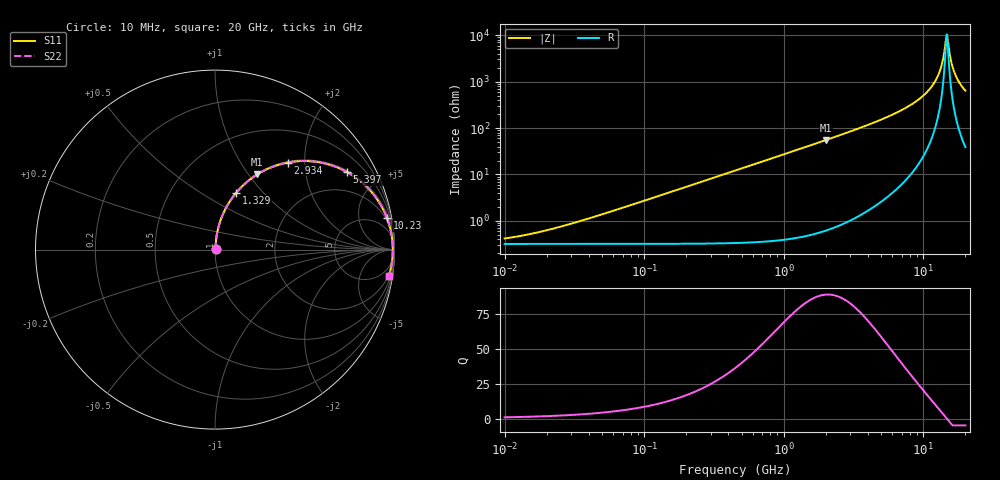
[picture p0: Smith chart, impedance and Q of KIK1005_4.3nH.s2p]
!version-3
!date-01.2023
!Series
# Hz S RI R 50
!Freq ReS11 ImS11 ReS21 ImS21 ReS12 ImS12 ReS22 ImS22
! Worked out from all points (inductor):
!   500 points, 10 MHz to 20 GHz, reference 50 ohm
!   read as one part in series: L = 4.3 nH near 35.95 MHz
!   highest Q = 89.2 at 2.005 GHz (marker M1), where L = 4.38 nH
!   self-resonance near 14.52 GHz
!   S11 on the Smith chart (normalised r, x): 10 MHz: 1.01, +0.01; 1.329 GHz: 1.01, +0.72; 2.934 GHz: 1.02, +1.65; 5.397 GHz: 1.06, +3.37; 10.23 GHz: 2, +11; 20 GHz: 2, -13
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1e7  0.00319 0.00268  0.9968 -0.00268  0.9968 -0.00268  0.00319 0.00268
3.59488e7  0.00328 0.00965  0.9967 -0.00965  0.9967 -0.00965  0.00328 0.00965
1.272781e8  0.00436 0.0341  0.9956 -0.0341  0.9956 -0.0341  0.00436 0.0341
4.506326e8  0.0178 0.1193  0.9822 -0.1193  0.9822 -0.1193  0.0178 0.1193
1.328949e9  0.1189 0.3175  0.8811 -0.3175  0.8811 -0.3175  0.1189 0.3175
1.595481e9  0.1627 0.3633  0.8373 -0.3633  0.8373 -0.3633  0.1627 0.3633
2.005031e9  0.236 0.4191  0.764 -0.4191  0.764 -0.4191  0.236 0.4191
2.934292e9  0.4064 0.4852  0.5936 -0.4852  0.5936 -0.4852  0.4064 0.4852
5.396535e9  0.7355 0.432  0.2645 -0.432  0.2645 -0.432  0.7355 0.432
5.648861e9  0.7577 0.4189  0.2423 -0.4189  0.2423 -0.4189  0.7577 0.4189
7.897639e9  0.8925 0.295  0.1075 -0.295  0.1075 -0.295  0.8925 0.295
1.023192e10  0.9574 0.1774  0.0426 -0.1774  0.0426 -0.1774  0.9574 0.1774
1.173532e10  0.9777 0.1115  0.0223 -0.1115  0.0223 -0.1115  0.9777 0.1115
1.285839e10  0.9859 0.0668  0.0141 -0.0668  0.0141 -0.0668  0.9859 0.0668
1.36662e10  0.9891 0.0368  0.0109 -0.0368  0.0109 -0.0368  0.9891 0.0368
1.452476e10  0.9904 0.00682  0.00958 -0.00682  0.00958 -0.00682  0.9904 0.00682
1.47477e10  0.9905 -0.000696  0.00953 0.000696  0.00953 0.000696  0.9905 -0.000696
1.497406e10  0.9904 -0.00821  0.00959 0.00821  0.00959 0.00821  0.9904 -0.00821
1.591478e10  0.989 -0.0382  0.011 0.0382  0.011 0.0382  0.989 -0.0382
1.665891e10  0.9868 -0.0607  0.0132 0.0607  0.0132 0.0607  0.9868 -0.0607
1.825317e10  0.9792 -0.1055  0.0208 0.1055  0.0208 0.1055  0.9792 -0.1055
2e10  0.9674 -0.1497  0.0326 0.1497  0.0326 0.1497  0.9674 -0.1497
